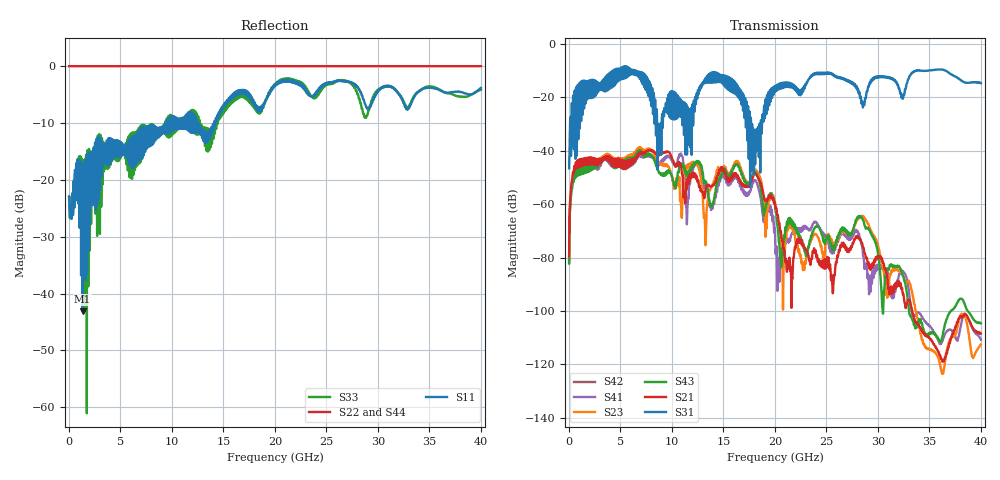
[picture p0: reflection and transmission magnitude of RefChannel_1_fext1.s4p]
# GHz S RI R 50
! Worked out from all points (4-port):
!   4000 points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, 10 MHz to 40 GHz, reference 50 ohm
!   strongest paths, dB at 10 MHz, 10.01 GHz, 20.01 GHz, 30.01 GHz, 40 GHz:
!     S31: -46.6, -28.1, -18.0, -12.3, -14.7
!     S21: -79.5, -43.0, -59.9, -80.2, -108.5
!     S43: -82.2, -49.9, -60.8, -78.6, -104.6
!     S23: -81.9, -49.7, -59.8, -75.5, -112.6
!     S41: -80.9, -43.8, -70.4, -84.2, -110.7
!     S42: -, -, -, -, -
!   lowest |S11| = -43.1 dB at 1.31 GHz (marker M1), VSWR 1.01, Z = 50.3 + j0.652 ohm
!   |S11| at or under -10 dB: start of sweep to 9.465 GHz; 12.43 GHz to 12.53 GHz (103.5 MHz wide, 0.829 % of centre); 12.55 GHz to 14.09 GHz (1.537 GHz wide, 11.5 % of centre)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
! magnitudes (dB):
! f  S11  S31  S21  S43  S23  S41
! 10 MHz  -22.9  -46.6  -79.5  -82.2  -81.9  -80.9
! 1.31 GHz  -43.1  -22.4  -44.1  -46.7  -45.6  -45.3
! 8.78 GHz  -11.3  -36.3  -41.7  -48.1  -44.6  -44.4
! 14.53 GHz  -8.2  -11.2  -48.8  -51.0  -47.1  -53.1
! 18.02 GHz  -6.3  -32.4  -48.8  -48.0  -47.2  -51.1
! 20.78 GHz  -2.7  -15.0  -75.0  -77.4  -99.5  -77.1
! 40 GHz  -3.8  -14.7  -108.5  -104.6  -112.6  -110.7
